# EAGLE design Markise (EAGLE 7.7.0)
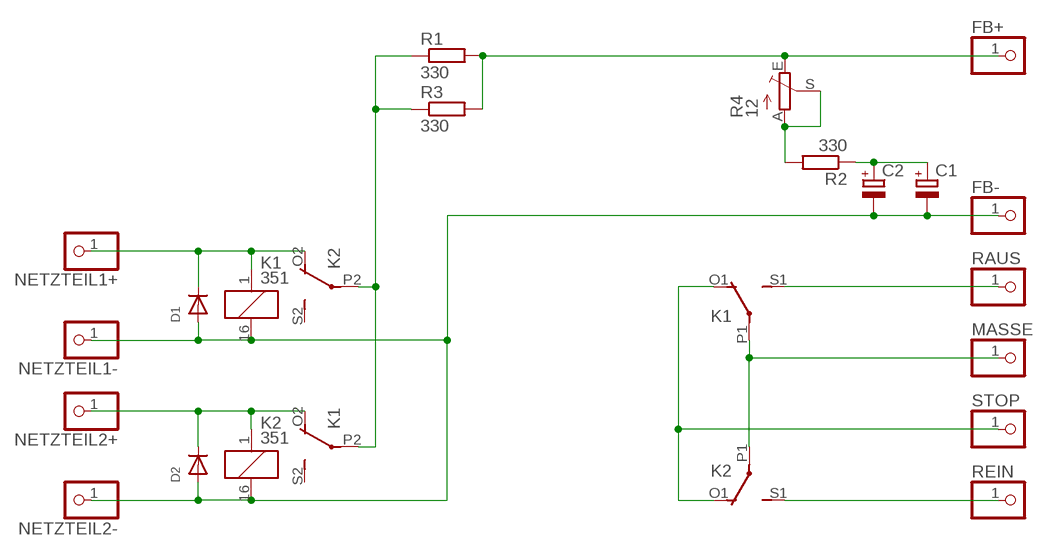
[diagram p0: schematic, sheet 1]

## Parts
C1  C-POL_RADIAL-11MM-DIA  [CAPPRD508W65D1000H1100B]
C2  C-POL_RADIAL-11MM-DIA  [CAPPRD508W65D1000H1100B]
D1  DIODEDO-1N4148  [DO-1N4148]
D2  DIODEDO-1N4148  [DO-1N4148]
FB+  PINHD-1X1  [1X01]
FB-  PINHD-1X1  [1X01]
K1  351  [351]
K2  351  [351]
MASSE  PINHD-1X1  [1X01]
NETZTEIL1+  PINHD-1X1  [1X01]
NETZTEIL1-  PINHD-1X1  [1X01]
NETZTEIL2+  PINHD-1X1  [1X01]
NETZTEIL2-  PINHD-1X1  [1X01]
R1  330  R-EU_0207/10  [0207/10]
R2  330  R-EU_0207/10  [0207/10]
R3  330  R-EU_0207/10  [0207/10]
R4  12  TRIM_EU-CIP20C-4MM  [CIP20C-4MM]
RAUS  PINHD-1X1  [1X01]
REIN  PINHD-1X1  [1X01]
STOP  PINHD-1X1  [1X01]

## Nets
GND: C1.2(-) C2.2(-) D1.A D2.A FB-.1 K1.16 K2.16 NETZTEIL1-.1 NETZTEIL2-.1
N$1: D1.C K1.1 K2.O2(3:O) NETZTEIL1+.1
N$2: C1.1(+) C2.1(+) R2.1
N$3: D2.C K1.O2(3:O) K2.1 NETZTEIL2+.1
N$4: R2.2 R4.A R4.S
N$5: K1.S1(2:S) RAUS.1
N$7: K1.P1(2:P) K2.P1(2:P) MASSE.1
N$8: K2.S1(2:S) REIN.1
N$9: K1.O1(2:O) K2.O1(2:O) STOP.1
N$10: FB+.1 R1.2 R3.2 R4.E
N$12: K1.P2(3:P) K2.P2(3:P) R1.1 R3.1
Unconnected: K1.S2(3:S) K2.S2(3:S)

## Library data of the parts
C1 C2 = Capacitor:C-POL: Capacitor Polarised - Generic; CATEGORY: Capacitor
D1 D2 = adafruit:DIODE: Diode
FB+ FB- MASSE NETZTEIL1+ NETZTEIL1- NETZTEIL2+ NETZTEIL2- RAUS REIN STOP = adafruit:PINHD-1X1: Pin header 1x1 for 0.1" spacing
K1 K2 = relay:351: RELAY 2 x switch, Omron; OC_FARNELL: unknown; OC_NEWARK: unknown
R1-R3 = resistor:R-EU_: RESISTOR, European symbol
R4 = pot:TRIM_EU-: POTENTIOMETER

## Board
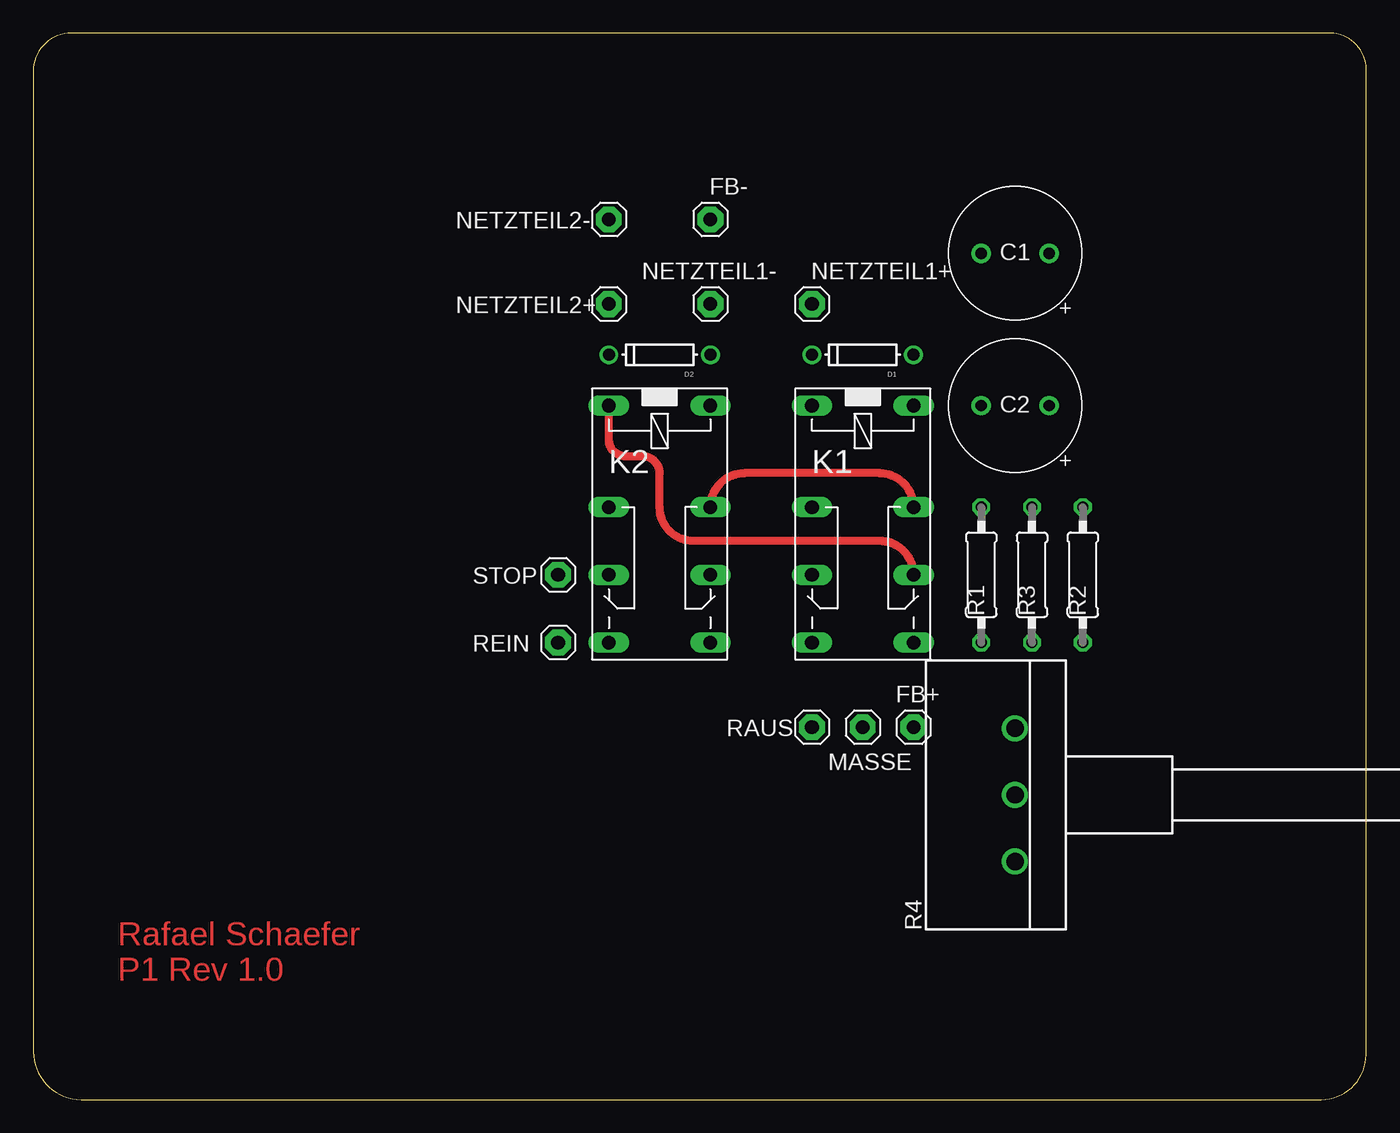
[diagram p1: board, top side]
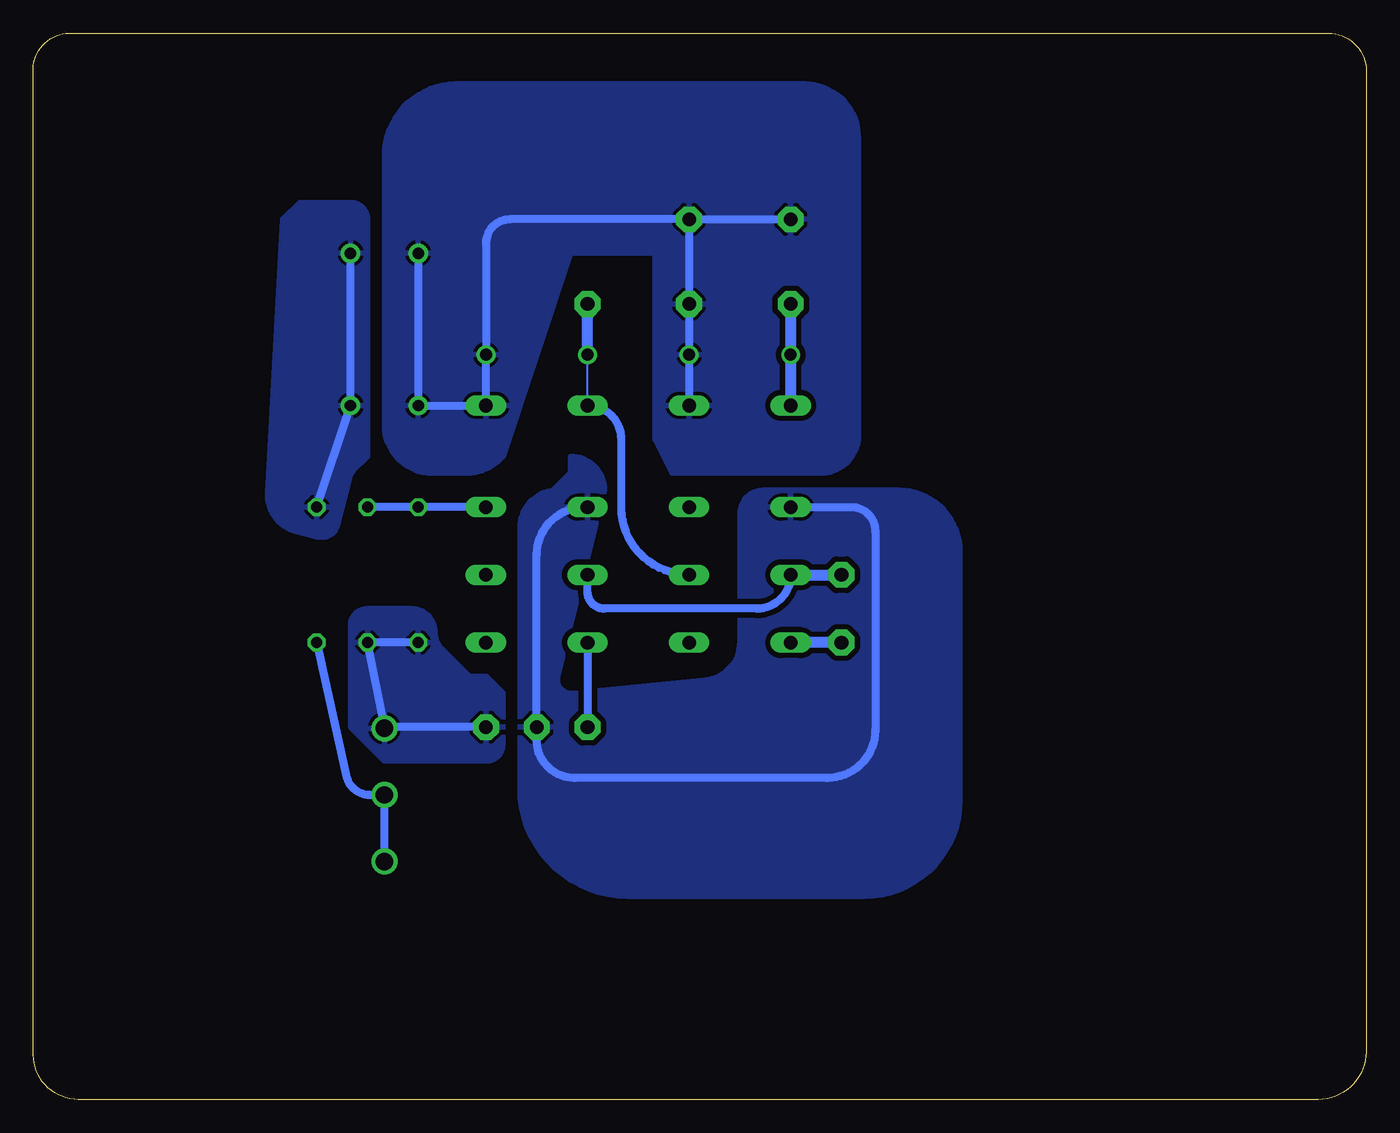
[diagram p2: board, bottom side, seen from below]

Size 100 x 80 mm. Coordinates in mm from the lower left corner, seen from the top.
Outline: 97.3,80 2.83,80 arc90 0,77.17 0,3.59 arc90 3.59,0 96.63,0 arc90 100,3.37 100,77.3 arc90 97.3,80
Copper layers (1*16): Top 0.035mm / dielectric 1.5mm / Bottom 0.035mm
Design rules "default *": minimum track width 16mil, minimum drill 0.35mm, track to track 6mil, track to pad 6mil, pad to pad 6mil, via to via 6mil, smd to smd 6mil, copper to edge 40mil, drill to drill 6mil, minimum pad ring 10mil, minimum via ring 8mil, stop-mask expansion 4mil, vias tented up to drill 0mil, thermal gap 10mil

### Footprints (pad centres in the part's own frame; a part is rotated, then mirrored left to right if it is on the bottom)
CAPPRD508W65D1000H1100B = drill 0.85 pad 1.45: 1 -2.54,0; 2 2.54,0
DO-1N4148 = drill 0.9: A -3.81,0; C 3.81,0
1X01 = drill 1.016 pad 1.93 octagon: 1 0,0
351 = drill 1.016 long: 1 -3.81,-3.81; 16 -3.81,3.81; O1 8.89,-3.81; O2 8.89,3.81; P1 3.81,-3.81; P2 3.81,3.81; S1 13.97,-3.81; S2 13.97,3.81
0207/10 = drill 0.813 octagon: 1 -5.08,0; 2 5.08,0
CIP20C-4MM = drill 1.3 pad 1.93: A -5,0; E 5,0; S 0,0

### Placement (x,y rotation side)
C1  73.66,63.5 180 top
C2  73.66,52.07 180 top
D1  62.23,55.88 180 top
D2  46.99,55.88 180 top
FB+  66.04,27.94 0 top
FB-  50.8,66.04 0 top
K1  62.23,48.26 270 top
K2  46.99,48.26 270 top
MASSE  62.23,27.94 0 top
NETZTEIL1+  58.42,59.69 0 top
NETZTEIL1-  50.8,59.69 0 top
NETZTEIL2+  43.18,59.69 0 top
NETZTEIL2-  43.18,66.04 0 top
R1  71.12,39.37 270 top
R2  78.74,39.37 270 top
R3  74.93,39.37 270 top
R4  73.66,22.86 90 top
RAUS  58.42,27.94 0 top
REIN  39.37,34.29 0 top
STOP  39.37,39.37 0 top

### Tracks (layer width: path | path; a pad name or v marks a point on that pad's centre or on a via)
GND
  Bottom 0.61: C1.2 C2.2 K1.16 D1.A 66.04,64.24 arc90 64.24,66.04 FB-.1 | K2.16 D2.A NETZTEIL1-.1 FB-.1 | FB-.1 NETZTEIL2-.1
  pour Bottom (isolate 0.406): 70.07,46.99 67.53,46.99 arc-45 64.99,48.04 64.77,48.26 59.69,63.5 53.34,63.5 53.34,49.53 52.07,46.99 40.94,46.99 arc-90 38.1,49.83 38.1,72.18 arc-90 42.12,76.2 68.27,76.2 arc-90 73.66,70.81 73.66,50.58 arc-90
N$1
  Bottom 0.152: K1.1 D1.C
  Bottom 0.61: K2.O2 arc90 55.88,44.45 55.88,49.53 arc-90 K1.1
  Bottom 0.813: D1.C NETZTEIL1+.1
N$2
  Bottom 0.61: C1.1 C2.1 R2.1
  pour Bottom: 80.01,67.31 76.2,67.31 arc90 74.93,66.04 74.93,48.26 75.95,47.24 arc-31 76.29,46.65 77.16,43.14 arc90 78.7,42.22 80.27,42.61 arc79 82.42,45.52 81.28,66.04
N$3
  Top 0.61: K1.O2 arc90 63.5,41.91 49.53,41.91 arc-90 46.99,44.45 46.99,46.99 arc90 45.72,48.26 44.45,48.26 arc-90 43.18,49.53 K2.1
  Bottom 0.813: NETZTEIL2+.1 D2.C K2.1
N$4
  Bottom 0.61: R2.2 76.51,24.27 arc-77 74.76,22.86 R4.S R4.A
N$5
  Bottom 0.61: K1.S1 RAUS.1
N$7
  Bottom 0.61: K1.P1 58.64,44.45 arc-90 62.23,40.86 MASSE.1 62.23,26.97 arc-90 59.39,24.13 40.42,24.13 arc-90 36.83,27.72 36.83,42.65 arc-90 38.63,44.45 K2.P1
  pour Bottom (isolate 0.406): 55.37,15.24 37.66,15.24 arc-90 30.48,22.42 30.48,41.14 arc-90 35.06,45.72 45.19,45.72 arc-90 46.99,43.92 46.99,34.32 arc84 49.55,31.49 59.69,30.48 arc104 60.65,31.71 57.15,45.72 arc-90 59.69,48.26 59.69,46.99 60.96,45.72 60.66,45.72 arc-90 63.5,42.88 63.5,23.37 arc-90
N$8
  Bottom 0.813: REIN.1 K2.S1
N$9
  Bottom 0.61: K2.O1 arc90 45.72,36.83 57.15,36.83 arc90 58.42,38.1 K1.O1
  Bottom 0.813: K2.O1 STOP.1
N$10
  Bottom 0.61: R1.2 R3.2 73.66,27.94 | R4.E 73.66,27.94 | FB+.1 73.66,27.94
  pour Bottom: 64.77,30.48 64.77,26.67 arc90 66.04,25.4 73.66,25.4 76.2,27.94 76.2,35.56 arc90 74.93,36.83 71.65,36.83 arc90 69.85,35.03 69.85,35.03 arc-45 69.32,33.76 67.31,31.75 66.04,31.75
N$12
  Top 0.61: K1.P2 arc90 63.5,46.99 53.34,46.99 arc90 K2.P2
  Bottom 0.61: 51.54,44.45 K2.P2 | K1.P2 R1.1 R3.1

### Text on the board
Top: Rafael Schaefer / P1 Rev 1.0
